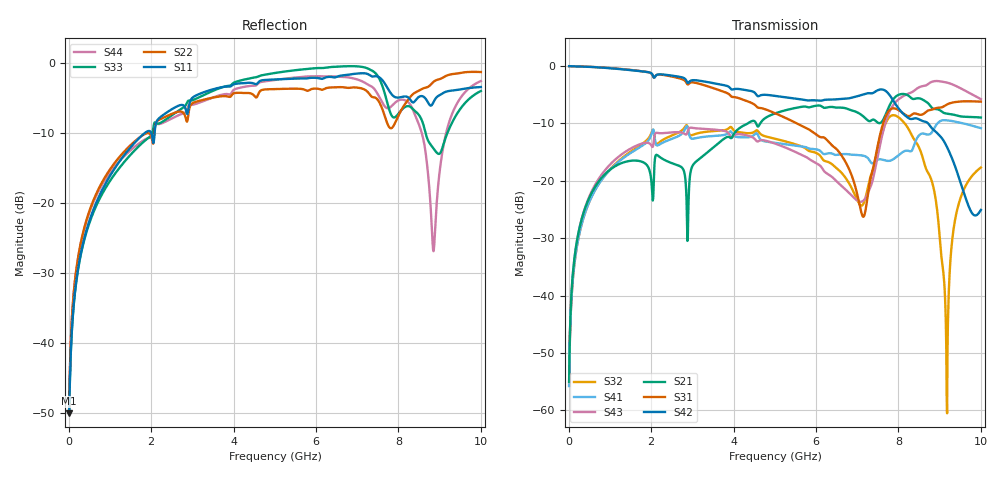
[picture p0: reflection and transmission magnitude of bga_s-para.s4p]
! Touchstone(R) file created by  Ansoft SIwave 8.0.0
! Touchstone(R) file created on Mon Jul 01 11:36:38 2013
! Port[1] = p1
! Port[2] = p2
! Port[3] = p3
! Port[4] = p4
! S-parameters
# Hz S MA R 50.000000
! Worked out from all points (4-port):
!   1000 points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, 10 MHz to 10 GHz, reference 50 ohm
!   strongest paths, dB at 10 MHz, 2.51 GHz, 5.01 GHz, 7.51 GHz, 10 GHz:
!     S42: 0.0, -1.7, -5.2, -4.2, -25.1
!     S31: 0.0, -1.8, -8.2, -13.4, -6.2
!     S21: -55.0, -16.9, -8.2, -9.9, -9.0
!     S43: -55.1, -11.6, -13.5, -15.2, -5.8
!     S41: -55.8, -12.7, -13.4, -16.3, -10.8
!     S32: -55.7, -12.1, -12.7, -14.4, -17.7
!   lowest |S11| = -50.0 dB at 10 MHz (marker M1), VSWR 1.01, Z = 50.3 + j0.159 ohm
!   |S11| at or under -10 dB: start of sweep to 1.846 GHz; 2.002 GHz to 2.084 GHz (81.32 MHz wide, 3.98 % of centre)
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1e7  0.003174 29.9  0.001773 61.8  0.9973 -0.4  0.001629 -120.7
     0.001773 61.8  0.003451 33.8  0.001638 -120.6  0.9971 -0.4
     0.9973 -0.4  0.001638 -120.6  0.003163 30.4  0.001759 61.9
     0.001629 -120.7  0.9971 -0.4  0.001759 61.9  0.003447 34.3
5.3e8  0.07902 45.2  0.07516 58.6  0.9841 -18.1  0.06944 -115.3
       0.07516 58.6  0.09271 48.9  0.06956 -115.2  0.9822 -19.0
       0.9841 -18.1  0.06956 -115.2  0.07615 84.1  0.0772 73.0
       0.06944 -115.3  0.9822 -19.0  0.0772 73.0  0.09055 79.9
2.02e9  0.3034 -58.4  0.08561 -39.3  0.8499 -71.2  0.2629 -177.2
        0.08561 -39.3  0.2869 -48.4  0.2685 -179.7  0.8547 -73.0
        0.8499 -71.2  0.2685 -179.7  0.3104 86.9  0.1993 37.0
        0.2629 -177.2  0.8547 -73.0  0.1993 37.0  0.2936 75.3
7.14e9  0.8445 110.4  0.3664 35.8  0.04874 -136.0  0.1658 7.9
        0.3664 35.8  0.6534 116.3  0.06218 63.1  0.565 148.1
        0.04874 -136.0  0.06218 63.1  0.9352 -3.1  0.06679 -99.2
        0.1658 7.9  0.565 148.1  0.06679 -99.2  0.7347 -1.7
7.99e9  0.566 89.5  0.5586 40.7  0.4158 -138.1  0.1658 168.7
        0.5586 40.7  0.4145 131.1  0.3604 12.5  0.4338 87.9
        0.4158 -138.1  0.3604 12.5  0.431 -3.6  0.5078 103.7
        0.1658 168.7  0.4338 87.9  0.5078 103.7  0.539 -0.3
9.17e9  0.6261 86.0  0.3851 0.1  0.4615 -169.5  0.3366 53.6
        0.3851 0.1  0.8127 106.7  0.001359 -76.4  0.1997 15.5
        0.4615 -169.5  0.001359 -76.4  0.3071 46.9  0.7185 9.9
        0.3366 53.6  0.1997 15.5  0.7185 9.9  0.3279 83.8
1e10  0.6735 66.0  0.356 -11.2  0.4896 159.3  0.2876 10.6
      0.356 -11.2  0.8619 80.6  0.1308 37.9  0.05581 -131.9
      0.4896 159.3  0.1308 37.9  0.6312 42.7  0.5148 -26.5
      0.2876 10.6  0.05581 -131.9  0.5148 -26.5  0.7437 52.6
